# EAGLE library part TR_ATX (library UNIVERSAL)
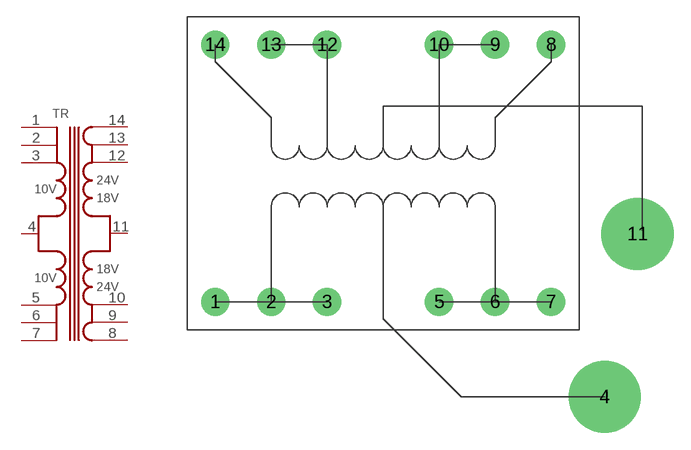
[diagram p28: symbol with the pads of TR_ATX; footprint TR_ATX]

Designator prefix TR

## TR_ATX  [TR_ATX]
1  1
2  2
3  3
4  4
5  5
6  6
7  7
8  8
9  9
10  10
11  11
12  12
13  13
14  14

## Footprint TR_ATX (pad centres in mm)
drill 1.1 pad 2.54: 1 2.5,2.5; 2 7.5,2.5; 3 12.5,2.5; 5 22.5,2.5; 6 27.5,2.5; 7 32.5,2.5; 8 32.5,25.5; 9 27.5,25.5; 10 22.5,25.5; 12 12.5,25.5; 13 7.5,25.5; 14 2.5,25.5
drill 2.8 pad 6.452: 4 37.29,-6; 11 40.23,8.57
